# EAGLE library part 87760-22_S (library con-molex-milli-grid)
HEADER
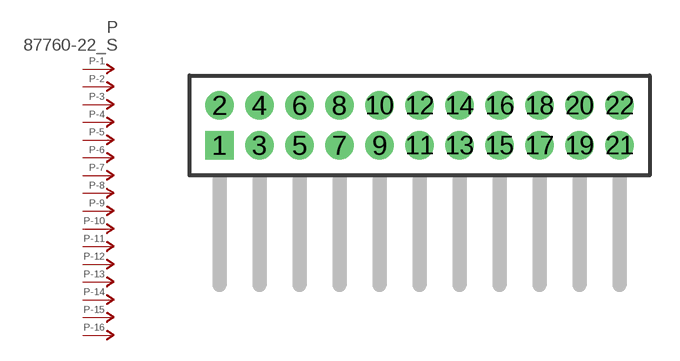
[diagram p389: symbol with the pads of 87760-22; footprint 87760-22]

Designator prefix P; gates -1=P-NV -2=P-N -3=P-N -4=P-N -5=P-N -6=P-N -7=P-N -8=P-N -9=P-N -10=P-N -11=P-N -12=P-N -13=P-N -14=P-N -15=P-N -16=P-N -17=P-N -18=P-N -19=P-N -20=P-N -21=P-N -22=P-N

## 87760-22_S  [87760-22]
1  -1:P  pas
2  -2:P  pas
3  -3:P  pas
4  -4:P  pas
5  -5:P  pas
6  -6:P  pas
7  -7:P  pas
8  -8:P  pas
9  -9:P  pas
10  -10:P  pas
11  -11:P  pas
12  -12:P  pas
13  -13:P  pas
14  -14:P  pas
15  -15:P  pas
16  -16:P  pas
17  -17:P  pas
18  -18:P  pas
19  -19:P  pas
20  -20:P  pas
21  -21:P  pas
22  -22:P  pas

## Footprint 87760-22 (pad centres in mm)
HEADER Dual Row, Right Angle
drill 0.914 square: 1 -10,-1
drill 0.914: 2 -10,1; 3 -8,-1; 4 -8,1; 5 -6,-1; 6 -6,1; 7 -4,-1; 8 -4,1; 9 -2,-1; 10 -2,1; 11 0,-1; 12 0,1; 13 2,-1; 14 2,1; 15 4,-1; 16 4,1; 17 6,-1; 18 6,1; 19 8,-1; 20 8,1; 21 10,-1; 22 10,1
